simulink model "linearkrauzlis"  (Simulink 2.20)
settings: Solver=ode45  StartTime=0.0  StopTime=2  RelTol=1e-3  AbsTol=1e-6

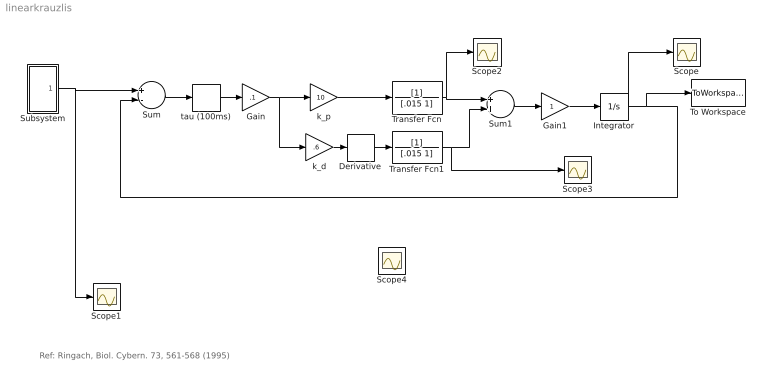
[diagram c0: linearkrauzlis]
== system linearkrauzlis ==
  note: Ref: Ringach, Biol. Cybern. 73, 561-568 (1995)
  Derivative : Derivative
  Gain : Gain  Gain=.1
  Gain1 : Gain  Gain=1
  Integrator : Integrator  ExternalReset=none  InitialConditionSource=internal  InitialCondition=0  LimitOutput=off  UpperSaturationLimit=inf  LowerSaturationLimit=-inf  ShowSaturationPort=off  ShowStatePort=off  AbsoluteTolerance=auto
  Scope{,1..4} (5 alike) : Scope
  Subsystem : Subsystem
  Sum : Sum  Inputs=+-
  Sum1 : Sum  Inputs=++
  To Workspace : ToWorkspace  VariableName=simout  SampleTime=.01
  Transfer Fcn : TransferFcn  Numerator=[1]  Denominator=[.015 1]
  Transfer Fcn1 : TransferFcn  Numerator=[1]  Denominator=[.015 1]
  k_d : Gain  Gain=.6
  k_p : Gain  Gain=10
  tau (100ms) : TransportDelay  DelayTime=80e-3  InitialInput=0  BufferSize=1024
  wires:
  Sum/1 -> tau (100ms)/1
  k_d/1 -> Derivative/1
  Integrator/1 -> Scope/1, Sum/2, To Workspace/1
  Subsystem/1(Out1) -> Sum/1, Scope1/1
  k_p/1 -> Transfer Fcn/1
  Derivative/1 -> Transfer Fcn1/1
  Transfer Fcn/1 -> Sum1/1, Scope2/1
  Transfer Fcn1/1 -> Sum1/2, Scope3/1
  tau (100ms)/1 -> Gain/1
  Gain/1 -> k_p/1, k_d/1
  Sum1/1 -> Gain1/1
  Gain1/1 -> Integrator/1

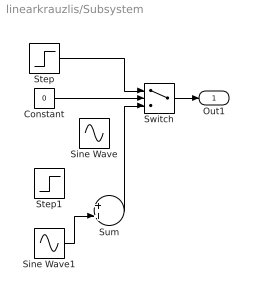
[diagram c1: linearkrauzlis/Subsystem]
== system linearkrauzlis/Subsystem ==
  Constant : Constant  Value=0
  Sine Wave : Sin  Amplitude=10  Frequency=10*pi*2  Phase=0  SampleTime=0
  Sine Wave1 : Sin  Amplitude=8  Frequency=6*pi*2  Phase=0  SampleTime=0
  Step : Step  Time=.1  Before=0  After=20
  Step1 : Step  Time=.1  Before=0  After=20
  Sum : Sum  Inputs=++
  Switch : Switch  Threshold=1
  Out1 : Outport  Port=1  InitialOutput=0
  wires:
  Constant/1 -> Switch/2
  Switch/1 -> Out1/1
  Sine Wave1/1 -> Sum/2
  Sum/1 -> Switch/3
  Step/1 -> Switch/1
